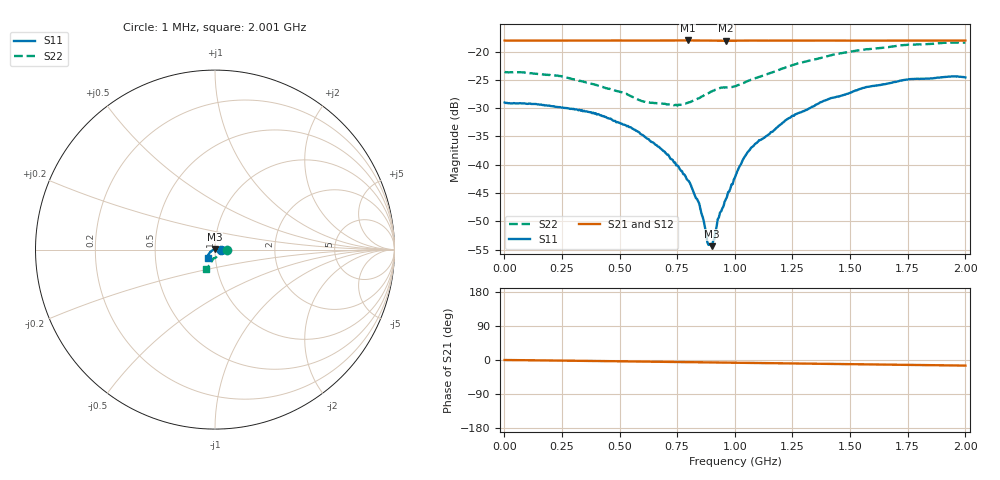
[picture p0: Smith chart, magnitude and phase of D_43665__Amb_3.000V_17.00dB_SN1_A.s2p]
! device id: 43665_
! dir: \\malibu\benchdata\1_engineers\tn_data\43665_75ohm\new\sparar\43665_\amb\3p000v\17p00db
! Serial: 1
! Insertion: A
! Temp: Amb
! VDD: 3.000V
! Attenuation Step: 17.00dB
! IDD: 1.442018e+00mA
! FILE NAME
! DATE 03-27-2009 08:37:31
! CORRECTED  DATA
#  Hz  S  RI  R  75
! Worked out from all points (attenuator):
!   401 points, 1 MHz to 2.001 GHz, reference 75 ohm
!   highest |S21| = -18.04 dB at 796 MHz (marker M1); lowest = -18.1 dB at 961 MHz (marker M2)
!   lowest |S11| = -54.4 dB at 901 MHz (marker M3), VSWR 1.00, Z = 74.8 + j0.165 ohm
!   |S11| at or under -10 dB: start of sweep to end of sweep
!   |S22| runs from -29.5 to -18.4 dB; largest |S21 - S12| = 0.00056
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1000000  0.0355 -0.000211  0.1251 -0.000111  0.1252 -8.9e-05  0.0661 -0.000726
2.36e8  0.032 0.00403  0.1249 -0.00335  0.125 -0.00333  0.0608 -0.00231
3.36e8  0.03 0.00532  0.1249 -0.00489  0.125 -0.00482  0.0543 -0.00426
5.46e8  0.0204 0.00658  0.1248 -0.00821  0.1249 -0.00812  0.0382 -0.0137
6.11e8  0.0165 0.00607  0.1247 -0.00917  0.1248 -0.00908  0.0315 -0.0173
6.71e8  0.0132 0.00566  0.1247 -0.0102  0.1248 -0.00997  0.0272 -0.0221
7.41e8  0.00926 0.00487  0.1247 -0.0114  0.1248 -0.0112  0.0208 -0.0265
7.96e8  0.00612 0.00395  0.1246 -0.0124  0.1247 -0.0122  0.0151 -0.0319
8.46e8  0.00285 0.00353  0.1245 -0.0134  0.1245 -0.0132  0.0104 -0.0374
8.86e8  -0.000451 0.00191  0.1242 -0.0142  0.1243 -0.014  0.0063 -0.0424
9.01e8  -0.00155 0.00111  0.124 -0.0145  0.1241 -0.0142  0.00439 -0.0443
9.36e8  -0.00378 -0.00014  0.1237 -0.015  0.1238 -0.0147  -0.00125 -0.0476
9.61e8  -0.00492 -0.000569  0.1235 -0.0151  0.1237 -0.0148  -0.00566 -0.0479
1.001e9  -0.00769 -0.00096  0.1237 -0.0154  0.1239 -0.0151  -0.00897 -0.0485
1.046e9  -0.0117 -0.00267  0.1239 -0.0163  0.1241 -0.016  -0.011 -0.0526
1.096e9  -0.0147 -0.0052  0.1238 -0.0174  0.124 -0.0171  -0.0135 -0.0572
1.241e9  -0.0235 -0.0113  0.1234 -0.0198  0.1237 -0.0196  -0.0219 -0.0713
1.336e9  -0.0282 -0.0163  0.1231 -0.0214  0.1235 -0.0211  -0.0277 -0.0796
1.546e9  -0.0375 -0.0282  0.1223 -0.025  0.1228 -0.0249  -0.0378 -0.096
1.671e9  -0.0397 -0.0343  0.1219 -0.027  0.1222 -0.0271  -0.0422 -0.1014
1.766e9  -0.0406 -0.0402  0.1216 -0.0285  0.122 -0.0287  -0.0442 -0.1064
2.001e9  -0.0377 -0.0455  0.1209 -0.0319  0.1208 -0.0322  -0.051 -0.1086
